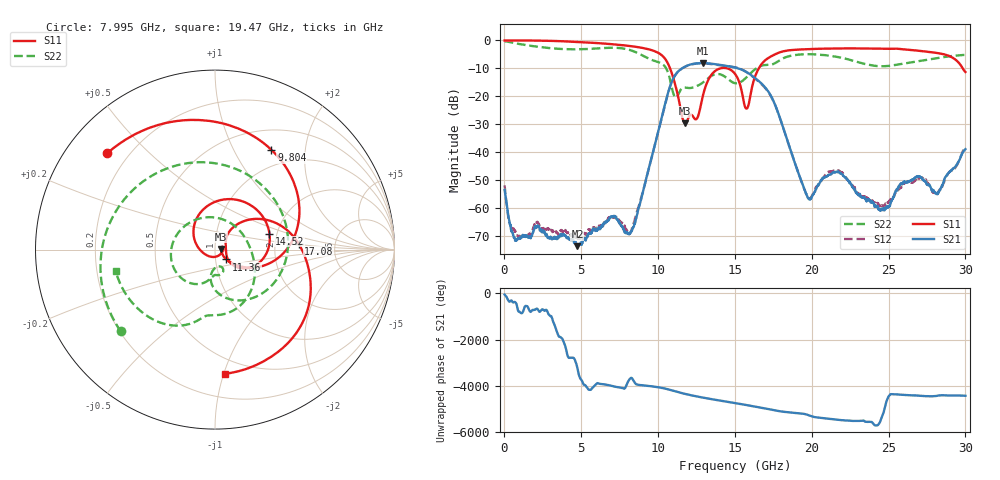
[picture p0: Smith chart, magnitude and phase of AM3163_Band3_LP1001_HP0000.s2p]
!Agilent Technologies,E8364B,MY43040894,A.07.50.67
!Agilent E8364B: A.07.50.67
!Date: Thursday, August 20, 2020 12:12:01
!Correction: S11(Full 2 Port(1,2))
!S21(Full 2 Port(1,2))
!S12(Full 2 Port(1,2))
!S22(Full 2 Port(1,2))
!S2P File: Measurements: S11, S21, S12, S22:
# Hz S  dB  R 50
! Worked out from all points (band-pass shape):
!   3201 points, 10 MHz to 30 GHz, reference 50 ohm
!   highest |S21| = -8.08 dB at 12.92 GHz (marker M1); lowest = -73.5 dB at 4.752 GHz (marker M2)
!   |S21| within 3 dB of the highest: 11.3 GHz to 15.69 GHz (4.383 GHz wide, 32.5 % of centre)
!   lowest |S11| = -29.6 dB at 11.77 GHz (marker M3), VSWR 1.07, Z = 53.4 + j0.396 ohm
!   |S11| at or under -10 dB: 10.78 GHz to 14.03 GHz (3.253 GHz wide, 26.2 % of centre); 14.52 GHz to 16.55 GHz (2.035 GHz wide, 13.1 % of centre); 29.83 GHz to end of sweep
!   |S22| runs from -20.4 to -0.3 dB; largest |S21 - S12| = 0.011
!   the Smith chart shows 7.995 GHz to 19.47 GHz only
!   S11 on the Smith chart (normalised r, x): 7.995 GHz: 0.12, +0.38; 9.804 GHz: 0.76, +1.43; 11.36 GHz: 1.13, -0.12; 14.52 GHz: 1.83, +0.36; 17.08 GHz: 2.73, +0.23; 19.47 GHz: 0.38, -1.01
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1e7  -0.01 -1.9  -53.45 -48.1  -51.74 -56.3  -0.27 -6.3
1.078394e9  -0.01 -29.6  -70.67 -131.8  -70.54 114.1  -1.38 -83.6
2.371712e9  -0.08 -65.0  -67.57 -27.2  -66.61 -20.6  -2.40 -163.8
4.752169e9  -0.53 -128.6  -73.51 -18.9  -70.59 -88.5  -3.17 69.8
5.014581e9  -0.60 -135.6  -73.02 -155.1  -70.21 48.5  -3.14 55.5
6.382875e9  -1.07 -172.8  -65.80 25.1  -66.13 28.0  -2.73 -24.6
7.994838e9  -1.88 138.2  -68.53 63.6  -68.10 -141.5  -3.16 -139.1
9.044488e9  -2.73 98.5  -53.36 -25.7  -53.38 -26.6  -5.54 122.8
9.803609e9  -3.90 60.5  -37.01 -88.1  -37.03 -88.5  -7.36 33.9
1.000979e10  -4.43 47.7  -32.53 -109.1  -32.60 -109.8  -7.73 7.4
1.135934e10  -21.48 -40.7  -10.80 27.1  -10.83 27.2  -18.68 -67.4
1.17717e10  -29.58 6.4  -9.30 -40.3  -9.36 -40.3  -16.86 -83.6
1.291507e10  -19.75 167.3  -8.08 162.2  -8.16 162.0  -15.03 -102.8
1.451766e10  -10.00 16.3  -9.15 -20.4  -9.17 -18.9  -13.64 135.2
1.5005e10  -11.93 -17.7  -9.68 -74.3  -9.58 -73.5  -15.28 67.5
1.577349e10  -24.34 8.5  -11.36 -163.6  -11.38 -164.1  -13.04 -14.7
1.707618e10  -6.62 4.1  -17.53 37.7  -17.71 39.3  -8.75 -88.8
1.946601e10  -3.17 -85.2  -52.28 -178.1  -52.39 -173.2  -4.95 -167.6
2.000958e10  -3.03 -99.8  -55.94 65.9  -55.48 74.0  -4.93 173.0
2.215574e10  -2.84 -149.9  -48.80 -107.8  -48.52 -110.9  -6.45 89.4
2.500479e10  -2.98 144.2  -59.50 -140.6  -57.76 -79.1  -9.12 -63.8
3e10  -11.28 -31.0  -38.85 -118.9  -37.87 -117.1  -5.15 108.1
